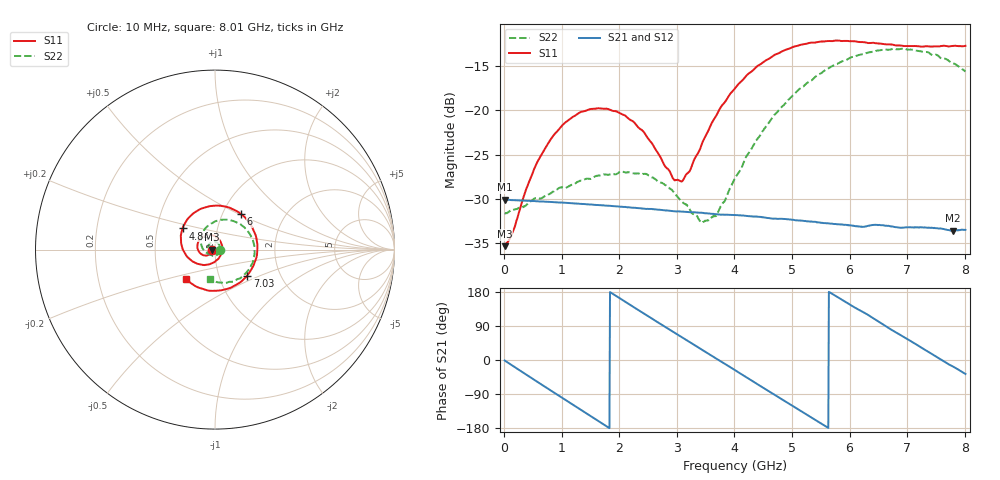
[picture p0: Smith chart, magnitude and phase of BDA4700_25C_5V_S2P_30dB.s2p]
!Agilent Technologies,E5071B,MY42404982,A.09.10
!Date: Mon Oct 20 13:41:42 2025
!Data & Calibration Information:
!Freq	S11:SOLT2(ON)	S21:SOLT2(ON)	S12:SOLT2(ON)	S22:SOLT2(ON)
# Hz S RI R 50
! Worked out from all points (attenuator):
!   801 points, 10 MHz to 8.01 GHz, reference 50 ohm
!   highest |S21| = -30.05 dB at 10 MHz (marker M1); lowest = -33.6 dB at 7.8 GHz (marker M2)
!   lowest |S11| = -35.3 dB at 10 MHz (marker M3), VSWR 1.03, Z = 48.3 - j0.101 ohm
!   |S11| at or under -10 dB: start of sweep to end of sweep
!   |S22| runs from -32.7 to -13.0 dB; largest |S21 - S12| = 0.00029
!   S11 on the Smith chart (normalised r, x): 10 MHz: 0.97, -0.00; 4.84 GHz: 0.68, +0.17; 6 GHz: 1.21, +0.52; 7.03 GHz: 1.36, -0.42; 8.01 GHz: 0.69, -0.24
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1e7  -0.0171 -0.00104  0.0314 -0.000637  0.0314 -0.000678  0.0263 -0.000821
1.5e8  -0.0182 -0.00962  0.0301 -0.00817  0.0301 -0.00823  0.0265 -0.00718
6.3e8  -0.0438 -0.0329  0.0141 -0.0272  0.0141 -0.0273  0.0108 -0.03
1.01e9  -0.079 -0.0233  -0.00521 -0.0297  -0.00521 -0.0297  -0.0153 -0.0336
1.35e9  -0.098 0.00845  -0.0203 -0.0216  -0.0203 -0.0217  -0.036 -0.0178
2.08e9  -0.0489 0.0806  -0.0261 0.0116  -0.0262 0.0116  -0.0299 0.0335
2.68e9  0.0278 0.0497  -0.00414 0.0272  -0.00412 0.0273  0.0127 0.0375
2.95e9  0.0397 0.00885  0.0079 0.0258  0.00787 0.0258  0.0252 0.0234
3.1e9  0.0367 -0.0161  0.0139 0.023  0.0138 0.023  0.028 0.0116
3.41e9  0.00664 -0.0609  0.023 0.0131  0.0231 0.0131  0.0206 -0.0114
3.54e9  -0.0136 -0.0747  0.0251 0.00782  0.0251 0.00781  0.0131 -0.0202
3.7e9  -0.0454 -0.0838  0.0259 0.00105  0.026 0.000972  -0.000496 -0.026
4.01e9  -0.1115 -0.0728  0.0229 -0.0116  0.023 -0.0116  -0.0321 -0.0259
4.43e9  -0.1803 0.00283  0.00992 -0.023  0.0099 -0.0231  -0.0702 0.00994
4.84e9  -0.1808 0.1182  -0.00643 -0.0236  -0.00635 -0.0237  -0.0764 0.0733
5.35e9  -0.0723 0.2297  -0.021 -0.0106  -0.0211 -0.0107  -0.0155 0.1479
6e9  0.1429 0.1999  -0.0188 0.0124  -0.0189 0.0124  0.1309 0.1472
6.68e9  0.2344 -0.0232  0.00231 0.0222  0.0023 0.0222  0.2197 0.000492
7.03e9  0.1794 -0.1445  0.0132 0.0175  0.0133 0.0174  0.1992 -0.0932
7.44e9  0.044 -0.2245  0.0211 0.00548  0.021 0.00542  0.1163 -0.1686
7.8e9  -0.0964 -0.2098  0.0199 -0.00639  0.02 -0.00649  0.0208 -0.183
8.01e9  -0.163 -0.1636  0.017 -0.0127  0.017 -0.0127  -0.0301 -0.1626
